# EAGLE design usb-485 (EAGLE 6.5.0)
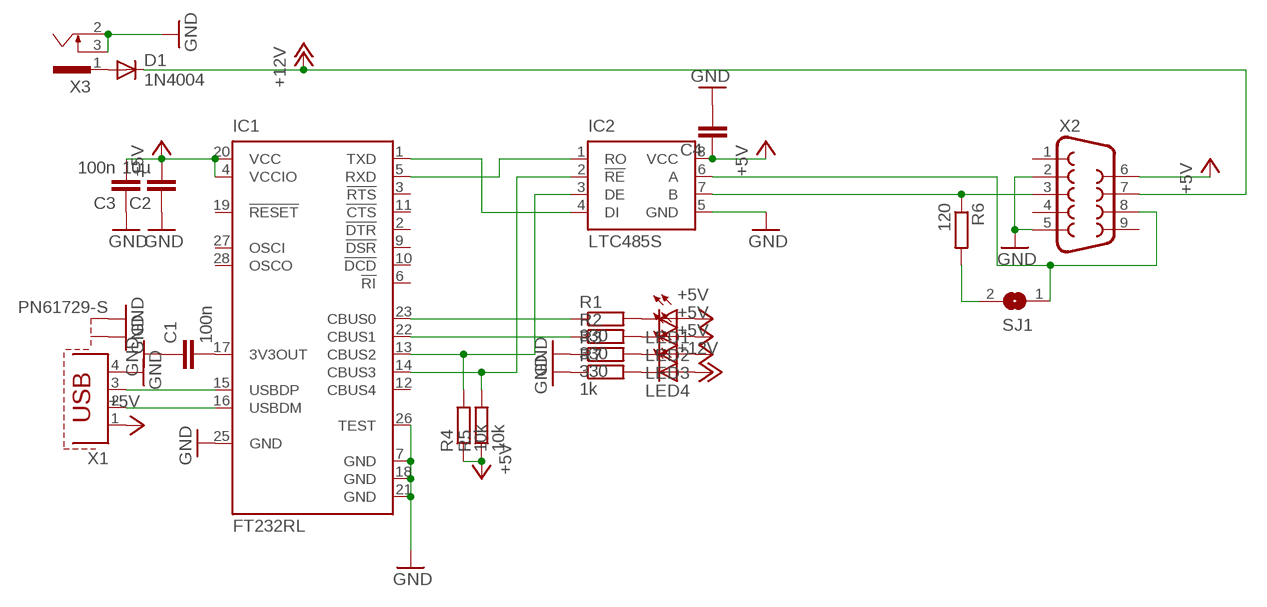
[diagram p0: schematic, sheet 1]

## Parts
C1  100n  C-EUC0805  [C0805]
C2  10µ  C-EUC0805  [C0805]
C3  100n  C-EUC0805  [C0805]
C4  C-EUC0805  [C0805]
D1  1N4004  [DO41-10]
IC1  FT232RL  [SSOP28]
IC2  LTC485S  [SOIC8]
LED1  LED3MM  [LED3MM]
LED2  LED3MM  [LED3MM]
LED3  LED3MM  [LED3MM]
LED4  LED3MM  [LED3MM]
R1  330  R-EU_M0805  [M0805]
R2  330  R-EU_M0805  [M0805]
R3  330  R-EU_M0805  [M0805]
R4  10k  R-EU_M0805  [M0805]
R5  10k  R-EU_M0805  [M0805]
R6  120  R-EU_M0805  [M0805]
R7  1k  R-EU_M0805  [M0805]
SJ1  SJ  [SJ]
X1  PN61729-S  [PN61729-S]
X2  F09HP  [F09HP]
X3  733980-62  [733980-62]

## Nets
+5V: C2.2 C3.2 C4.1 IC1.4(VCCIO) IC1.20(VCC) IC2.8(VCC) LED1.A LED2.A LED3.A R4.1 R5.1 X1.1 X2.6
+12V: D1.C LED4.A X2.7
GND: C1.1 C2.1 C3.1 C4.2 IC1.7(GND) IC1.18(GND) IC1.21(GND) IC1.25(GND) IC1.26(TEST) IC2.5(GND) R3.1 R7.1 X1.4 X1.S1 X1.S2 X2.2 X2.5 X3.2 X3.3
N$1: IC2.7(B) R6.1 X2.3
N$2: IC2.6(A) SJ1.1 X2.8
N$3: R6.2 SJ1.2
N$5: IC1.1(TXD) IC2.4(DI)
N$6: IC1.5(RXD) IC2.1(RO)
N$7: IC1.14(CBUS3) IC2.2(!RE) R5.2
N$8: IC1.13(CBUS2) IC2.3(DE) R4.2
N$9: IC1.22(CBUS1) R2.1
N$10: IC1.23(CBUS0) R1.1
N$11: IC1.16(USBDM) X1.2
N$12: IC1.15(USBDP) X1.3
N$13: C1.2 IC1.17(3V3OUT)
N$14: LED1.K(C) R1.2
N$15: LED2.K(C) R2.2
N$16: LED3.K(C) R3.2
N$19: LED4.K(C) R7.2
N$20: D1.A X3.1
Unconnected: IC1.2(!DTR) IC1.3(!RTS) IC1.6(!RI) IC1.9(!DSR) IC1.10(!DCD) IC1.11(!CTS) IC1.12(CBUS4) IC1.19(!RESET) IC1.27(OSCI) IC1.28(OSCO) X2.1 X2.4 X2.9

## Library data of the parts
C1-C4 = rcl:C-EU: CAPACITOR, European symbol
D1 = diode:1N4004: DIODE
IC1 = ftdichip:FT232R: Source: http://www.ftdichip.com/Documents/DataSheets/DS_FT232R_v104.pdf; MPN: FT232RL; OC_FARNELL: 1146032; OC_NEWARK: 91K9918
IC2 = linear-technology:LTC485: Low Power RS485 Interface Transceiver Source: http://www.linear.com/pc/downloadDocument.do?navId=H0,C1,C1007,C1017,P2064,D1718; OC_FARNELL: unknown; OC_NEWARK: unknown
LED1-LED4 = led:LED: LED
R1-R7 = rcl:R-EU_: RESISTOR, European symbol
SJ1 = jumper:SJ: SMD solder JUMPER
X1 = con-berg:PN61729-S: BERG USB connector; OC_FARNELL: unknown; OC_NEWARK: unknown
X2 = con-subd:F09: SUB-D; OC_FARNELL: unknown; OC_NEWARK: unknown
X3 = con-conrad:73398?: FEMALE PRINT CONNECTOR Niedervolt-Steckverbinder Distributor Conrad

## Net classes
0 default: width 0.25 mm, drill 0 mm, clearance 0.2 mm

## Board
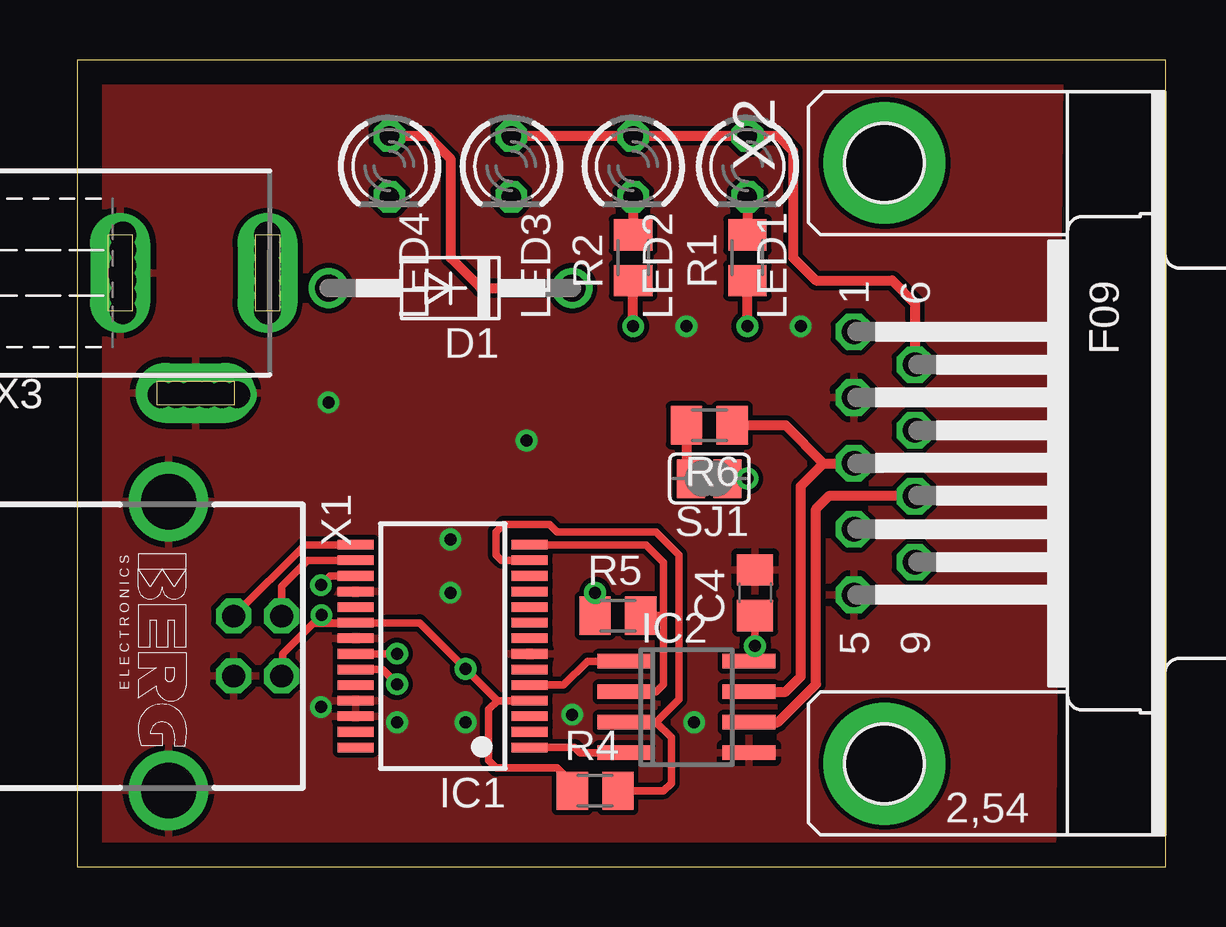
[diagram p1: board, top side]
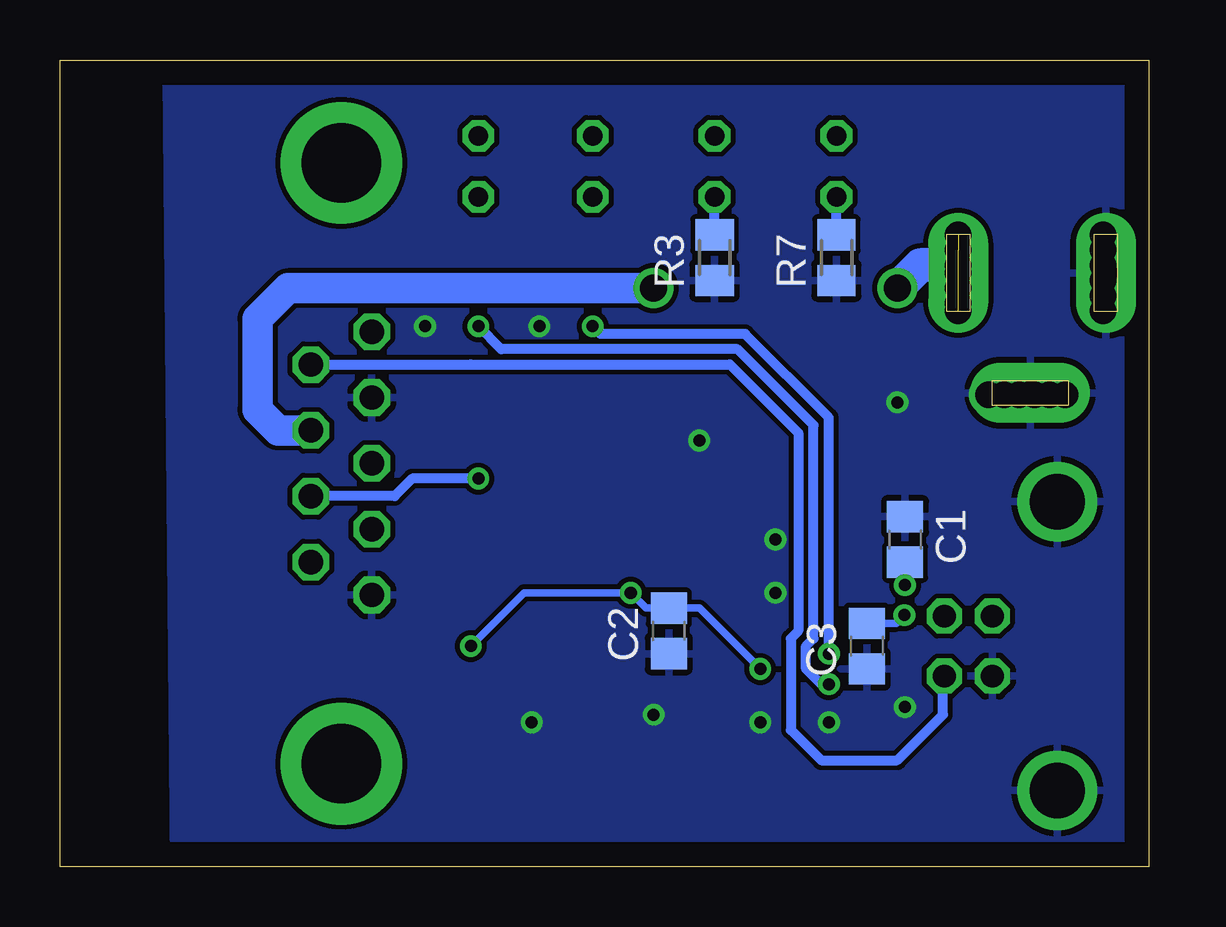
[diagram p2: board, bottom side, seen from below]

Size 45.38 x 33.64 mm. Coordinates in mm from the lower left corner, seen from the top.
Outline: 0,0 45.38,0 45.38,33.64 0,33.64 0,0
Copper layers (1*16): Top 0.035mm / dielectric 1.5mm / Bottom 0.035mm
Design rules "default": minimum track width 10mil, minimum drill 24mil, track to track 8mil, track to pad 8mil, pad to pad 8mil, via to via 8mil, smd to smd 8mil, copper to edge 40mil, drill to drill 8mil, minimum pad ring 10mil, minimum via ring 8mil, stop-mask expansion 4mil, vias tented up to drill 0mil, thermal gap 10mil

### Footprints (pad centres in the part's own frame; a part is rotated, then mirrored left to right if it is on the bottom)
C0805 = smd 1.3 x 1.5: 1 -0.95,0; 2 0.95,0
DO41-10 = drill 1.118: A 5.08,0; C -5.08,0
SSOP28 = smd 0.4 x 1.5: 1 -4.225,-3.625; 2 -3.575,-3.625; 3 -2.925,-3.625; 4 -2.275,-3.625; 5 -1.625,-3.625; 6 -0.975,-3.625; 7 -0.325,-3.625; 8 0.325,-3.625; 9 0.975,-3.625; 10 1.625,-3.625; 11 2.275,-3.625; 12 2.925,-3.625; 13 3.575,-3.625; 14 4.225,-3.625; 15 4.225,3.625; 16 3.575,3.625; 17 2.925,3.625; 18 2.275,3.625; 19 1.625,3.625; 20 0.975,3.625; 21 0.325,3.625; 22 -0.325,3.625; 23 -0.975,3.625; 24 -1.625,3.625; 25 -2.275,3.625; 26 -2.925,3.625; 27 -3.575,3.625; 28 -4.225,3.625
SOIC8 = smd 0.6 x 2.2: 1 -1.905,-2.6; 2 -0.635,-2.6; 3 0.635,-2.6; 4 1.905,-2.6; 5 1.905,2.6; 6 0.635,2.6; 7 -0.635,2.6; 8 -1.905,2.6
LED3MM = drill 0.813 octagon: A -1.27,0; K 1.27,0
M0805 = smd 1.3 x 1.6: 1 -0.95,0; 2 0.95,0
SJ = smd 1.168 x 1.6: 1 -0.762,0; 2 0.762,0
PN61729-S = drill 0.95 octagon: 1 1.25,4.71; 2 -1.25,4.71; 3 -1.25,2.71; 4 1.25,2.71 | drill 2.3 pad 2.9: S1 -6.02,0; S2 6.02,0
F09HP = drill 1.016 octagon: 1 -5.486,-1.27; 2 -2.743,-1.27; 3 0,-1.27; 4 2.743,-1.27; 5 5.486,-1.27; 6 -4.115,1.27; 7 -1.372,1.27; 8 1.372,1.27; 9 4.115,1.27 | drill 3.302 pad 5.08: G1 -12.522,0; G2 12.522,0
733980-62 = drill 1 pad 2.5 long: 1 0,8.57; 2 0,2.42; 3 5,5.57

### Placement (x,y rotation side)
C1  10.16,13.65 270 bottom
C2  20,9.84 90 bottom
C3  11.75,9.21 90 bottom
C4  28.26,11.43 90 top
D1  15.56,24.13 180 top
IC1  15.24,9.21 90 top
IC2  25.4,6.67 270 top
LED1  27.94,29.21 270 top
LED2  23.18,29.21 270 top
LED3  18.1,29.21 270 top
LED4  13.02,29.21 270 top
R1  27.94,25.4 90 top
R2  23.18,25.4 90 top
R3  18.1,25.4 90 bottom
R4  21.59,3.17 0 top
R5  22.54,10.48 0 top
R6  26.35,18.41 180 top
R7  13.02,25.4 90 bottom
SJ1  26.35,16.19 180 top
X1  3.81,9.21 270 top
X2  33.66,16.83 270 top
X3  -0.64,24.77 270 top

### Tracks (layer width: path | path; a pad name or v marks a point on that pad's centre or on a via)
+5V  (via drill 0.5)
  Top 0.305: IC1.20 10.79,10.18 | X1.1 8.57,8.01 8.57,8.89 9.84,10.16 10.79,10.16 11.59,10.16 IC1.20 | IC1.20 14.27,10.18 v16.19,8.26 17.52,6.93 | IC1.4 17.52,6.93 | 17.52,6.93 17.14,6.56 17.14,4.45 17.46,4.13 20,4.13 20.95,3.17 R4.1 20.64,2.54 | IC2.8 28.26,8.83 v28.26,9.21 C4.1 | R5.1 v21.59,11.43 | IC1.20 10.5,10.18 v10.18,10.5
  Top 0.406: LED3.A LED2.A LED1.A 29.21,30.48 29.84,29.84 29.84,25.4 30.8,24.45 33.97,24.45 34.92,23.5 X2.6
  Bottom 0.305: C2.2 18.73,10.79 v16.19,8.26 | v28.26,9.21 26.04,11.43 v21.59,11.43 20.96,10.79 C2.2 | C2.2 | C3.2 10.53,10.16 v10.18,10.5
  Bottom 0.406: X2.6 28.25,20.94 28.26,20.95 17.46,20.95 14.61,18.1 14.61,9.84 14.92,9.53 14.92,5.71 13.65,4.45 10.48,4.45 8.57,6.35 8.57,7.91 X1.1
+12V
  Top 0.406: LED4.A 14.61,30.48 15.56,29.53 15.56,25.4 16.83,24.13 D1.C
  Bottom 1.27: D1.C 35.88,24.13 37.15,22.86 37.15,19.05 36.3,18.2 X2.7
GND  (via drill 0.5, 1.1)
  other vias: 15.56,13.65 10.16,6.67 15.56,11.43 10.48,19.37 20.64,6.35 6.67,19.68 6.03,19.68 5.4,19.68 4.76,19.68 4.13,19.68 3.49,19.68 1.91,23.18 1.91,23.81 1.91,24.45 1.91,25.08 1.91,25.72 1.91,26.35 25.4,22.54 13.34,6.03 16.19,6.03 25.72,6.03 18.73,17.78 30.16,22.54
  pour Top: 0,0 0.32,33.02 40.96,33.02 40.64,0
  pour Bottom: 0.32,33.02 40.96,33.02 40.64,0 0,0
N$1
  Top 0.406: IC2.7 29.53,7.3 30.16,7.94 30.16,15.88 31.11,16.83 | 31.11,16.83 X2.3 | R6.1 29.53,18.41 31.11,16.83
N$2  (via drill 0.5)
  Top 0.406: IC2.6 29.21,6.03 30.8,7.62 30.8,14.92 31.33,15.46 X2.8 | SJ1.1 v27.94,16.19
  Bottom 0.406: v27.94,16.19 30.7,16.19 31.43,15.46 X2.8
N$3
  Top 0.406: R6.2 25.4,16.38 SJ1.2
N$5
  Top 0.305: IC1.1 20.73,4.98 20.95,4.76 IC2.4
N$6
  Top 0.305: IC1.5 20.28,7.58 21.27,8.57 IC2.1
N$7
  Top 0.305: IC2.2 24.13,7.3 24.45,7.62 24.45,10.48 | 24.45,10.48 24.45,12.7 23.71,13.43 IC1.14 | R5.2 24.45,10.48
N$8
  Top 0.305: IC2.3 24.13,6.03 | 24.13,6.03 25.08,6.99 25.08,13.02 24.13,13.97 20,13.97 19.68,14.29 17.78,14.29 17.46,13.97 17.46,13.02 17.7,12.78 IC1.13 | R4.2 24.45,3.17 24.77,3.49 24.77,5.4 24.13,6.03
N$9  (via drill 0.5)
  Top 0.305: IC1.22 13.33,8.88
  Top 0.406: 13.33,8.88 v13.34,8.89 | v23.18,22.54 R2.1
  Bottom 0.406: v13.34,8.89 13.34,18.73 16.83,22.23 22.86,22.23 v23.18,22.54
N$10  (via drill 0.5)
  Top 0.305: IC1.23 12.72,8.23 v13.34,7.62
  Top 0.406: v27.94,22.54 R1.1
  Bottom 0.406: v13.34,7.62 13.65,7.62 14.29,8.26 14.29,9.21 13.97,9.53 13.97,18.41 17.14,21.59 26.99,21.59 v27.94,22.54
N$11
  Top 0.305: IC1.16 9.61,12.78 8.52,11.7 X1.2
N$12
  Top 0.305: IC1.15 9.49,13.43 X1.3
N$13  (via drill 0.5)
  Top 0.305: IC1.17 10.54,12.13 v10.16,11.75
  Bottom 0.305: v10.16,11.75 C1.2 10.16,13.02
N$14
  Top 0.406: LED1.K R1.2
N$15
  Top 0.406: LED2.K R2.2
N$16
  Bottom 0.406: R3.2 LED3.K
N$19
  Bottom 0.406: R7.2 LED4.K
N$20  (via drill 1.1)  (7 unrouted)
  Bottom 1.422: v7.94,25.08 9.53,25.08 D1.A
  other vias: 7.94,24.77 7.94,25.72 7.94,26.35 7.94,24.13 7.94,23.5 7.94,23.18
